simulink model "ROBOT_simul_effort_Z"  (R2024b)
settings: Solver=VariableStepAuto  StartTime=0.0  StopTime=5  RelTol=1e-3
undefined symbols (not defined in the file): a, ARRIERE_Defaut_sldprt, avant01_Defaut_sldprt, avant02_Defaut_sldprt, avant03_Defaut_sldprt, avant1_Defaut_sldprt, AXE, BASE_Defaut_sldprt, BIELLE, BIELLE_Defaut_sldprt, BRAS_Defaut_sldprt, bras_Defaut_sldprt, C_Realiste_sldprt, CABLE_Defaut_sldprt, cable_Defaut_sldprt, CACHE_Defaut_sldprt, CARTE, carte_Defaut_sldprt, CARTER, carter, CHC, CODEUR_Defaut_sldprt, cruciforme, cylindrique, deg, Drive, Fichiers, Fichiers_Matlab_sujetA, FIXATION, fixation_Defaut_sldprt, H, HEXAGONALE_Defaut_sldprt, joint_Defaut_sldprt, kg, m, M4, M4_Defaut_sldprt, manette1_Defaut_sldprt, manette2_Defaut_sldprt, MATLAB, Matlab, matlab_Defaut_sldprt, mm, modif, MOTEUR_Defaut_sldprt, N, NEZ_Defaut_sldprt, nom, palier, PARALLELOGRAMME_Defaut_sldprt, petite, plaque, rad, Ressort, Rondelle, ROTOR_Defaut_sldprt, s, SET, simple, socle_Defaut_sldprt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
libraries: sm_lib x463, fl_lib x45, nesl_utility x27, simulink x2
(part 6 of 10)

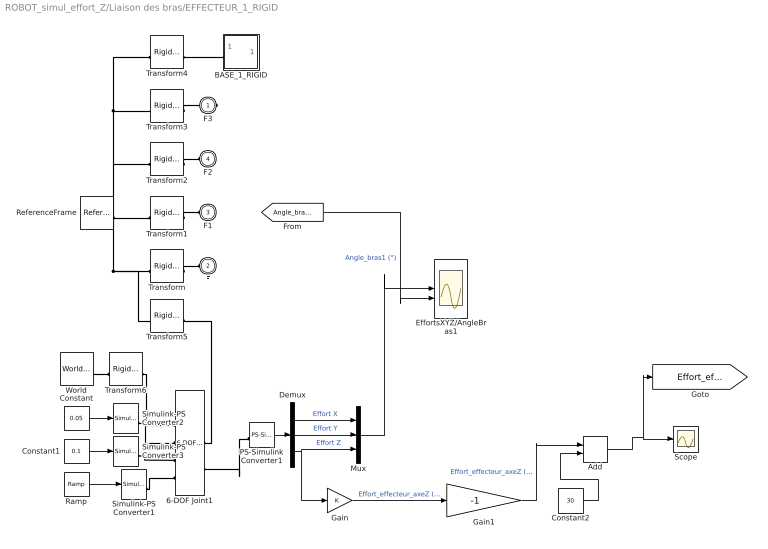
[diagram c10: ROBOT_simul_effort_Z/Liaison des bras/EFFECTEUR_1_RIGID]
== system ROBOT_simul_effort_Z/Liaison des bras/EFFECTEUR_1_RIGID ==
  6-DOF Joint1 : sm_lib/Joints/6-DOF Joint  JointMode=Normal  CompositeWrenchDir=FollowerOnBase  CompositeWrenchFrame=BaseFrame  SenseConstraintForce=off  SenseConstraintTorque=off  SenseTotalForce=on  SenseTotalTorque=off  PxPositionTargetSpecify=off  PxPositionTargetPriority=High  PxPositionTargetValue=0  PxPositionTargetValueUnits=m  PxVelocityTargetSpecify=off  PxVelocityTargetPriority=High  PxVelocityTargetValue=0  PxVelocityTargetValueUnits=m/s  PxEquilibriumPosition=0  PxEquilibriumPositionUnits=m  PxSpringStiffness=0  PxSpringStiffnessUnits=N/m  PxDampingCoefficient=0  PxDampingCoefficientUnits=N/(m/s)  PxLowerLimitSpecify=off  PxLowerLimitBound=-1  PxLowerLimitBoundUnits=m  PxLowerLimitStiffness=1e6  PxLowerLimitStiffnessUnits=N/m  PxLowerLimitDamping=1e3  PxLowerLimitDampingUnits=N/(m/s)  PxLowerLimitTransitionRegionWidth=1e-4  PxLowerLimitTransitionRegionWidthUnits=m  PxUpperLimitSpecify=off  PxUpperLimitBound=1  PxUpperLimitBoundUnits=m  PxUpperLimitStiffness=1e6  PxUpperLimitStiffnessUnits=N/m  PxUpperLimitDamping=1e3  PxUpperLimitDampingUnits=N/(m/s)  PxUpperLimitTransitionRegionWidth=1e-4  PxUpperLimitTransitionRegionWidthUnits=m  PxTorqueActuationMode=ComputedTorque  PxMotionActuationMode=InputMotion  PxSensePosition=off  PxSenseVelocity=off  PxSenseAcceleration=off  PxSenseTorqueForce=off  PxSenseLowerLimitTorqueForce=off  PxSenseUpperLimitTorqueForce=off  PyPositionTargetSpecify=off  PyPositionTargetPriority=High  PyPositionTargetValue=0  PyPositionTargetValueUnits=m  PyVelocityTargetSpecify=off  PyVelocityTargetPriority=High  PyVelocityTargetValue=0  PyVelocityTargetValueUnits=m/s  PyEquilibriumPosition=0  PyEquilibriumPositionUnits=m  PySpringStiffness=0  PySpringStiffnessUnits=N/m  PyDampingCoefficient=0  PyDampingCoefficientUnits=N/(m/s)  PyLowerLimitSpecify=off  PyLowerLimitBound=-1  PyLowerLimitBoundUnits=m  PyLowerLimitStiffness=1e6  PyLowerLimitStiffnessUnits=N/m  PyLowerLimitDamping=1e3  PyLowerLimitDampingUnits=N/(m/s)  PyLowerLimitTransitionRegionWidth=1e-4  PyLowerLimitTransitionRegionWidthUnits=m  PyUpperLimitSpecify=off  PyUpperLimitBound=1  PyUpperLimitBoundUnits=m  PyUpperLimitStiffness=1e6  PyUpperLimitStiffnessUnits=N/m  PyUpperLimitDamping=1e3  PyUpperLimitDampingUnits=N/(m/s)  PyUpperLimitTransitionRegionWidth=1e-4  PyUpperLimitTransitionRegionWidthUnits=m  PyTorqueActuationMode=ComputedTorque  PyMotionActuationMode=InputMotion  PySensePosition=off  PySenseVelocity=off  PySenseAcceleration=off  PySenseTorqueForce=off  PySenseLowerLimitTorqueForce=off  PySenseUpperLimitTorqueForce=off  PzPositionTargetSpecify=off  PzPositionTargetPriority=High  PzPositionTargetValue=0  PzPositionTargetValueUnits=m  PzVelocityTargetSpecify=off  PzVelocityTargetPriority=High  PzVelocityTargetValue=0  PzVelocityTargetValueUnits=m/s  PzEquilibriumPosition=0  PzEquilibriumPositionUnits=m  PzSpringStiffness=0  PzSpringStiffnessUnits=N/m  PzDampingCoefficient=0  PzDampingCoefficientUnits=N/(m/s)  PzLowerLimitSpecify=off  PzLowerLimitBound=-1  PzLowerLimitBoundUnits=m  PzLowerLimitStiffness=1e6  PzLowerLimitStiffnessUnits=N/m  PzLowerLimitDamping=1e3  PzLowerLimitDampingUnits=N/(m/s)  PzLowerLimitTransitionRegionWidth=1e-4  PzLowerLimitTransitionRegionWidthUnits=m  PzUpperLimitSpecify=off  PzUpperLimitBound=1  PzUpperLimitBoundUnits=m  PzUpperLimitStiffness=1e6  PzUpperLimitStiffnessUnits=N/m  PzUpperLimitDamping=1e3  PzUpperLimitDampingUnits=N/(m/s)  PzUpperLimitTransitionRegionWidth=1e-4  PzUpperLimitTransitionRegionWidthUnits=m  PzTorqueActuationMode=ComputedTorque  PzMotionActuationMode=InputMotion  PzSensePosition=off  PzSenseVelocity=off  PzSenseAcceleration=off  PzSenseTorqueForce=off  PzSenseLowerLimitTorqueForce=off  PzSenseUpperLimitTorqueForce=off  SphPositionTargetSpecify=off  SphPositionTargetPriority=High  SphPositionTargetRotationMethod=None  SphPositionTargetFollAlignAxisA=+X  SphPositionTargetBaseAlignAxisA=+Y  SphPositionTargetFollAlignAxisB=+Y  SphPositionTargetBaseAlignAxisB=+Z  SphPositionTargetRotationStandardAxis=+Z  SphPositionTargetRotationAngle=0.0  SphPositionTargetRotationAngleUnits=deg  SphPositionTargetRotationArbitraryAxis=[0 0 1]  SphPositionTargetRotationSequenceAxes=FollowerAxes  SphPositionTargetRotationSequence=XYX  SphPositionTargetRotationSequenceAngles=[0 0 0]  SphPositionTargetRotationSequenceAnglesUnits=deg  SphPositionTargetRotationMatrix=[1 0 0; 0 1 0; 0 0 1]  SphPositionTargetQuaternion=[1 0 0 0]  SphVelocityTargetSpecify=off  SphVelocityTargetPriority=High  SphVelocityTargetValue=[0 0 0]  SphVelocityTargetValueUnits=deg/s  SphVelocityTargetInFollowerFrame=on  SphEqPosRotationMethod=None  SphEqPosFollAlignAxisA=+X  SphEqPosBaseAlignAxisA=+Y  SphEqPosFollAlignAxisB=+Y  SphEqPosBaseAlignAxisB=+Z  SphEqPosRotationStandardAxis=+Z  SphEqPosRotationAngle=0.0  SphEqPosRotationAngleUnits=deg  SphEqPosRotationArbitraryAxis=[0 0 1]  SphEqPosRotationSequenceAxes=FollowerAxes  SphEqPosRotationSequence=XYX  SphEqPosRotationSequenceAngles=[0 0 0]  SphEqPosRotationSequenceAnglesUnits=deg  SphEqPosRotationMatrix=[1 0 0; 0 1 0; 0 0 1]  SphEqPosQuaternion=[1 0 0 0]  SphSpringStiffness=0  SphSpringStiffnessUnits=N*m/deg  SphDampingCoefficient=0  SphDampingCoefficientUnits=N*m/(deg/s)  SphLowerLimitSpecify=off  SphLowerLimitBound=15  SphLowerLimitBoundUnits=deg  SphLowerLimitStiffness=1e4  SphLowerLimitStiffnessUnits=N*m/deg  SphLowerLimitDamping=10  SphLowerLimitDampingUnits=N*m/(deg/s)  SphLowerLimitTransitionRegionWidth=0.1  SphLowerLimitTransitionRegionWidthUnits=deg  SphUpperLimitSpecify=off  SphUpperLimitBound=45  SphUpperLimitBoundUnits=deg  SphUpperLimitStiffness=1e4  SphUpperLimitStiffnessUnits=N*m/deg  SphUpperLimitDamping=10  SphUpperLimitDampingUnits=N*m/(deg/s)  SphUpperLimitTransitionRegionWidth=0.1  SphUpperLimitTransitionRegionWidthUnits=deg  SphTorqueActuationMode=NoTorque  SphActuateTorqueX=off  SphActuateTorqueY=off  SphActuateTorqueZ=off  SphActuateTorque=off  SphActuationFrame=BaseFrame  SphSensePosition=off  SphSenseVelocityX=off  SphSenseVelocityY=off  SphSenseVelocityZ=off  SphSenseVelocity=off  SphSenseAccelerationX=off  SphSenseAccelerationY=off  SphSenseAccelerationZ=off  SphSenseAcceleration=off  SphSenseLowerLimitTorqueMag=off  SphSenseUpperLimitTorqueMag=off  SphSensingFrame=BaseFrame
  Add : Sum
  BASE_1_RIGID : Subsystem
  Constant : Constant  Value=0.05
  Constant1 : Constant  Value=0.1
  Constant2 : Constant  Value=30
  Demux : Demux  Outputs=3
  EffortsXYZ/AngleBras1 : Scope  NumInputPorts=2
  Gain : Gain
  Gain1 : Gain  Gain=-1
  Mux : Mux  Inputs=3
  PS-Simulink Converter1 : nesl_utility/PS-Simulink Converter  PhysicalDomain=network_engine_domain  SubClassName=ps_output  LeftPortType=input  RightPortType=output  PseudoPeriodic=off  Frequencies=[]  VectorFormat=1-D array  Unit=1  AffineConversion=off
  Ramp : simulink/Sources/Ramp  slope=-0.022  start=0  InitialOutput=0.097
  ReferenceFrame : sm_lib/Frames and Transforms/Reference Frame
  Scope : Scope
  Simulink-PS Converter1 : nesl_utility/Simulink-PS Converter  PhysicalDomain=network_engine_domain  SubClassName=ps_input  LeftPortType=input  RightPortType=output  PseudoPeriodic=off  Frequencies=[]  NoiseDistribution=none  NoiseParameters=[]  Unit=m  AffineConversion=off  FilteringAndDerivatives=filter  SimscapeFilterOrder=2  InputFilterTimeConstant=0.0001  UdotUserProvided=1
  Simulink-PS Converter2 : nesl_utility/Simulink-PS Converter  PhysicalDomain=network_engine_domain  SubClassName=ps_input  LeftPortType=input  RightPortType=output  PseudoPeriodic=off  Frequencies=[]  NoiseDistribution=none  NoiseParameters=[]  Unit=m  AffineConversion=off  FilteringAndDerivatives=filter  SimscapeFilterOrder=2  InputFilterTimeConstant=0.0001  UdotUserProvided=1
  Simulink-PS Converter3 : nesl_utility/Simulink-PS Converter  PhysicalDomain=network_engine_domain  SubClassName=ps_input  LeftPortType=input  RightPortType=output  PseudoPeriodic=off  Frequencies=[]  NoiseDistribution=none  NoiseParameters=[]  Unit=m  AffineConversion=off  FilteringAndDerivatives=filter  SimscapeFilterOrder=2  InputFilterTimeConstant=0.0001  UdotUserProvided=1
  Transform : sm_lib/Frames and Transforms/Rigid Transform  RotationMethod=ArbitraryAxis  FollAlignAxisA=+X  BaseAlignAxisA=+Y  FollAlignAxisB=+Y  BaseAlignAxisB=+Z  RotationStandardAxis=+Z  RotationAngle=1.730474842144561  RotationAngleUnits=rad  RotationArbitraryAxis=[0.85183585180135124 0.37038876979862273 0.37038876979861218]  RotationSequenceAxes=FollowerAxes  RotationSequence=XYX  RotationSequenceAngles=[0 0 0]  RotationSequenceAnglesUnits=deg  RotationMatrix=[1 0 0; 0 1 0; 0 0 1]  Quaternion=[1 0 0 0]  TranslationMethod=Cartesian  TranslationCartesianOffset=[-87.428721422199686 114.78475141038592 178.68957730413138]  TranslationCartesianOffsetUnits=mm  TranslationStandardAxis=+Z  TranslationStandardOffset=0  TranslationStandardOffsetUnits=mm  TranslationROffset=0  TranslationROffsetUnits=m  TranslationThetaOffset=0  TranslationThetaOffsetUnits=deg  TranslationZOffset=0  TranslationZOffsetUnits=m
  Transform1 : sm_lib/Frames and Transforms/Rigid Transform  RotationMethod=ArbitraryAxis  FollAlignAxisA=+X  BaseAlignAxisA=+Y  FollAlignAxisB=+Y  BaseAlignAxisB=+Z  RotationStandardAxis=+Z  RotationAngle=2.2299847707569485  RotationAngleUnits=rad  RotationArbitraryAxis=[-0.6163079985177109 -0.49023351775065482 -0.61630799851771478]  RotationSequenceAxes=FollowerAxes  RotationSequence=XYX  RotationSequenceAngles=[0 0 0]  RotationSequenceAnglesUnits=deg  RotationMatrix=[1 0 0; 0 1 0; 0 0 1]  Quaternion=[1 0 0 0]  TranslationMethod=Cartesian  TranslationCartesianOffset=[-45.597843791303056 49.588932155076364 178.68957730412913]  TranslationCartesianOffsetUnits=mm  TranslationStandardAxis=+Z  TranslationStandardOffset=0  TranslationStandardOffsetUnits=mm  TranslationROffset=0  TranslationROffsetUnits=m  TranslationThetaOffset=0  TranslationThetaOffsetUnits=deg  TranslationZOffset=0  TranslationZOffsetUnits=m
  Transform2 : sm_lib/Frames and Transforms/Rigid Transform  RotationMethod=ArbitraryAxis  FollAlignAxisA=+X  BaseAlignAxisA=+Y  FollAlignAxisB=+Y  BaseAlignAxisB=+Z  RotationStandardAxis=+Z  RotationAngle=2.2733724201793901  RotationAngleUnits=rad  RotationArbitraryAxis=[-0.46360505726599749 -0.62652627673442052 0.62652627673442052]  RotationSequenceAxes=FollowerAxes  RotationSequence=XYX  RotationSequenceAngles=[0 0 0]  RotationSequenceAnglesUnits=deg  RotationMatrix=[1 0 0; 0 1 0; 0 0 1]  Quaternion=[1 0 0 0]  TranslationMethod=Cartesian  TranslationCartesianOffset=[-11.168668790429919 124.06200864616406 178.68957730412961]  TranslationCartesianOffsetUnits=mm  TranslationStandardAxis=+Z  TranslationStandardOffset=0  TranslationStandardOffsetUnits=mm  TranslationROffset=0  TranslationROffsetUnits=m  TranslationThetaOffset=0  TranslationThetaOffsetUnits=deg  TranslationZOffset=0  TranslationZOffsetUnits=m
  Transform3 : sm_lib/Frames and Transforms/Rigid Transform  RotationMethod=ArbitraryAxis  FollAlignAxisA=+X  BaseAlignAxisA=+Y  FollAlignAxisB=+Y  BaseAlignAxisB=+Z  RotationStandardAxis=+Z  RotationAngle=pi  RotationAngleUnits=rad  RotationArbitraryAxis=[-1 0 0]  RotationSequenceAxes=FollowerAxes  RotationSequence=XYX  RotationSequenceAngles=[0 0 0]  RotationSequenceAnglesUnits=deg  RotationMatrix=[1 0 0; 0 1 0; 0 0 1]  Quaternion=[1 0 0 0]  TranslationMethod=Cartesian  TranslationCartesianOffset=[-18.52 120.86 192.69]  TranslationCartesianOffsetUnits=mm  TranslationStandardAxis=+Z  TranslationStandardOffset=0  TranslationStandardOffsetUnits=mm  TranslationROffset=0  TranslationROffsetUnits=m  TranslationThetaOffset=0  TranslationThetaOffsetUnits=deg  TranslationZOffset=0  TranslationZOffsetUnits=m
  Transform4 : sm_lib/Frames and Transforms/Rigid Transform  RotationMethod=ArbitraryAxis  FollAlignAxisA=+X  BaseAlignAxisA=+Y  FollAlignAxisB=+Y  BaseAlignAxisB=+Z  RotationStandardAxis=+Z  RotationAngle=0.13705421065001749  RotationAngleUnits=rad  RotationArbitraryAxis=[5.1539164000577042e-14 1.7402105179219416e-14 -1]  RotationSequenceAxes=FollowerAxes  RotationSequence=XYX  RotationSequenceAngles=[0 0 0]  RotationSequenceAnglesUnits=deg  RotationMatrix=[1 0 0; 0 1 0; 0 0 1]  Quaternion=[1 0 0 0]  TranslationMethod=Cartesian  TranslationCartesianOffset=[-48.809383170568495 97.91432372411964 187.1895773041295]  TranslationCartesianOffsetUnits=mm  TranslationStandardAxis=+Z  TranslationStandardOffset=0  TranslationStandardOffsetUnits=mm  TranslationROffset=0  TranslationROffsetUnits=m  TranslationThetaOffset=0  TranslationThetaOffsetUnits=deg  TranslationZOffset=0  TranslationZOffsetUnits=m
  Transform5 : sm_lib/Frames and Transforms/Rigid Transform  RotationMethod=ArbitraryAxis  FollAlignAxisA=+X  BaseAlignAxisA=+Y  FollAlignAxisB=+Y  BaseAlignAxisB=+Z  RotationStandardAxis=+Z  RotationAngle=pi  RotationAngleUnits=rad  RotationArbitraryAxis=[-1 0 0]  RotationSequenceAxes=FollowerAxes  RotationSequence=XYX  RotationSequenceAngles=[0 0 0]  RotationSequenceAnglesUnits=deg  RotationMatrix=[1 0 0; 0 1 0; 0 0 1]  Quaternion=[1 0 0 0]  TranslationMethod=Cartesian  TranslationCartesianOffset=[-18.52 120.86 192.69]  TranslationCartesianOffsetUnits=mm  TranslationStandardAxis=+Z  TranslationStandardOffset=0  TranslationStandardOffsetUnits=mm  TranslationROffset=0  TranslationROffsetUnits=m  TranslationThetaOffset=0  TranslationThetaOffsetUnits=deg  TranslationZOffset=0  TranslationZOffsetUnits=m
  Transform6 : sm_lib/Frames and Transforms/Rigid Transform  RotationMethod=ArbitraryAxis  FollAlignAxisA=+X  BaseAlignAxisA=+Y  FollAlignAxisB=+Y  BaseAlignAxisB=+Z  RotationStandardAxis=+Z  RotationAngle=pi  RotationAngleUnits=rad  RotationArbitraryAxis=[-1 0 0]  RotationSequenceAxes=FollowerAxes  RotationSequence=XYX  RotationSequenceAngles=[0 0 0]  RotationSequenceAnglesUnits=deg  RotationMatrix=[1 0 0; 0 1 0; 0 0 1]  Quaternion=[1 0 0 0]  TranslationMethod=Cartesian  TranslationCartesianOffset=[-18.52 120.86 192.69]  TranslationCartesianOffsetUnits=mm  TranslationStandardAxis=+Z  TranslationStandardOffset=0  TranslationStandardOffsetUnits=mm  TranslationROffset=0  TranslationROffsetUnits=m  TranslationThetaOffset=0  TranslationThetaOffsetUnits=deg  TranslationZOffset=0  TranslationZOffsetUnits=m
  World : sm_lib/Frames and Transforms/World Frame
  F3 : PMIOPort  Side=Right
  F : PMIOPort  Port=2  Side=Left
  F1 : PMIOPort  Port=3  Side=Left
  F2 : PMIOPort  Port=4  Side=Left
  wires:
  Ramp/1 -> Simulink-PS Converter1/1
  Demux/3 -> Gain/1, Mux/3  "Effort Z"
  Constant/1 -> Simulink-PS Converter2/1
  Constant1/1 -> Simulink-PS Converter3/1
  [Angle_bras1] -> EffortsXYZ/AngleBras1/2  "Angle_bras1 (°)"
  Mux/1 -> EffortsXYZ/AngleBras1/1
  Demux/1 -> Mux/1  "Effort X"
  Demux/2 -> Mux/2  "Effort Y"
  PS-Simulink Converter1/1 -> Demux/1
  Gain/1 -> Gain1/1  "Effort_effecteur_axeZ (N)"
  Gain1/1 -> Add/1  "Effort_effecteur_axeZ (N)"
  Add/1 -> [Effort_effecteur], Scope/1
  Constant2/1 -> Add/2
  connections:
  ReferenceFrame/RConn1 -- Transform5/LConn1 -- Transform/LConn1 -- Transform1/LConn1 -- Transform2/LConn1 -- Transform3/LConn1 -- Transform4/LConn1
  Transform/RConn1 -- F/RConn1
  Transform1/RConn1 -- F1/RConn1
  Transform2/RConn1 -- F2/RConn1
  Transform3/RConn1 -- F3/RConn1
  BASE_1_RIGID/LConn1 -- Transform4/RConn1
  Simulink-PS Converter1/RConn1 -- 6-DOF Joint1/LConn4
  6-DOF Joint1/RConn1 -- Transform5/RConn1
  Transform6/RConn1 -- 6-DOF Joint1/LConn1
  World/RConn1 -- Transform6/LConn1
  Simulink-PS Converter2/RConn1 -- 6-DOF Joint1/LConn2
  Simulink-PS Converter3/RConn1 -- 6-DOF Joint1/LConn3
  PS-Simulink Converter1/LConn1 -- 6-DOF Joint1/RConn2

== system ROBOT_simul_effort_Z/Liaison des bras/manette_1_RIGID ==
  ReferenceFrame : sm_lib/Frames and Transforms/Reference Frame
  Transform : sm_lib/Frames and Transforms/Rigid Transform  RotationMethod=ArbitraryAxis  FollAlignAxisA=+X  BaseAlignAxisA=+Y  FollAlignAxisB=+Y  BaseAlignAxisB=+Z  RotationStandardAxis=+Z  RotationAngle=2.2920311904365782  RotationAngleUnits=rad  RotationArbitraryAxis=[0.63063758405056181 -0.45231899713116352 0.63063758405056158]  RotationSequenceAxes=FollowerAxes  RotationSequence=XYX  RotationSequenceAngles=[0 0 0]  RotationSequenceAnglesUnits=deg  RotationMatrix=[1 0 0; 0 1 0; 0 0 1]  Quaternion=[1 0 0 0]  TranslationMethod=Cartesian  TranslationCartesianOffset=[-33.84478008900291 22.436374240911583 2.2257143640758983]  TranslationCartesianOffsetUnits=mm  TranslationStandardAxis=+Z  TranslationStandardOffset=0  TranslationStandardOffsetUnits=mm  TranslationROffset=0  TranslationROffsetUnits=m  TranslationThetaOffset=0  TranslationThetaOffsetUnits=deg  TranslationZOffset=0  TranslationZOffsetUnits=m
  Transform1 : sm_lib/Frames and Transforms/Rigid Transform  RotationMethod=ArbitraryAxis  FollAlignAxisA=+X  BaseAlignAxisA=+Y  FollAlignAxisB=+Y  BaseAlignAxisB=+Z  RotationStandardAxis=+Z  RotationAngle=3.1415926535897931  RotationAngleUnits=rad  RotationArbitraryAxis=[-0.15005935073897111 0.98867699035417955 -3.0703282687218866e-18]  RotationSequenceAxes=FollowerAxes  RotationSequence=XYX  RotationSequenceAngles=[0 0 0]  RotationSequenceAnglesUnits=deg  RotationMatrix=[1 0 0; 0 1 0; 0 0 1]  Quaternion=[1 0 0 0]  TranslationMethod=Cartesian  TranslationCartesianOffset=[-57.010083199545775 -8.8196659542755462 4.7257143640759303]  TranslationCartesianOffsetUnits=mm  TranslationStandardAxis=+Z  TranslationStandardOffset=0  TranslationStandardOffsetUnits=mm  TranslationROffset=0  TranslationROffsetUnits=m  TranslationThetaOffset=0  TranslationThetaOffsetUnits=deg  TranslationZOffset=0  TranslationZOffsetUnits=m
  Transform2 : sm_lib/Frames and Transforms/Rigid Transform  RotationMethod=None  FollAlignAxisA=+X  BaseAlignAxisA=+Y  FollAlignAxisB=+Y  BaseAlignAxisB=+Z  RotationStandardAxis=+Z  RotationAngle=0  RotationAngleUnits=deg  RotationArbitraryAxis=[0 0 1]  RotationSequenceAxes=FollowerAxes  RotationSequence=XYX  RotationSequenceAngles=[0 0 0]  RotationSequenceAnglesUnits=deg  RotationMatrix=[1 0 0; 0 1 0; 0 0 1]  Quaternion=[1 0 0 0]  TranslationMethod=Cartesian  TranslationCartesianOffset=[-33.322737031332075 20.894129352085105 2.2257143640758983]  TranslationCartesianOffsetUnits=mm  TranslationStandardAxis=+Z  TranslationStandardOffset=0  TranslationStandardOffsetUnits=mm  TranslationROffset=0  TranslationROffsetUnits=m  TranslationThetaOffset=0  TranslationThetaOffsetUnits=deg  TranslationZOffset=0  TranslationZOffsetUnits=m
  manette1_1_RIGID : Subsystem
  F : PMIOPort  Side=Right
  F1 : PMIOPort  Port=2  Side=Left
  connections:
  Transform/LConn1 -- ReferenceFrame/RConn1 -- Transform1/LConn1 -- Transform2/LConn1
  Transform/RConn1 -- F/RConn1
  Transform1/RConn1 -- F1/RConn1
  Transform2/RConn1 -- manette1_1_RIGID/LConn1

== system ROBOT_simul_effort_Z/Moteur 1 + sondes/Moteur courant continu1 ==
  note: Kv = 1.18e-1
  Frottement : fl_lib/Mechanical/Rotational Elements/Rotational Friction  brkwy_trq=2.43e-3 N*m  brkwy_vel=0.030296 rad/s  Col_trq=2.43e-3 N*m  visc_coef=2e-6 N*m/(rad/s)  w_specify=off  w_priority=None  w=0 rad/s  w_nominal_specify=off  w_nominal_value=1  w_nominal_unit=rad/s  t_specify=off  t_priority=None  t=0 N*m  t_nominal_specify=off  t_nominal_value=1  t_nominal_unit=N*m
  Inductance induit 35mH : fl_lib/Electrical/Electrical Elements/Inductor  l=35 mH  r=0 Ohm  g=1e-09 1/Ohm  i_specify=off  i_priority=None  i=0 A  i_nominal_specify=off  i_nominal_value=1  i_nominal_unit=A  v_specify=off  v_priority=None  v=0 V  v_nominal_specify=off  v_nominal_value=1  v_nominal_unit=V  i_L_specify=on  i_L_priority=High  i_L=0 A  i_L_nominal_specify=off  i_L_nominal_value=1  i_L_nominal_unit=A
  Inertie Je 10e-6 : fl_lib/Mechanical/Rotational Elements/Inertia  inertia=10e-6 kg*m^2  num_ports=foundation.enum.numPorts2.one  w_specify=on  w_priority=High  w=0 rad/s  w_nominal_specify=off  w_nominal_value=1  w_nominal_unit=rad/s  t_specify=off  t_priority=None  t=0 N*m  t_nominal_specify=off  t_nominal_value=1  t_nominal_unit=N*m
  Moteur parfait : fl_lib/Electrical/Electrical Elements/Rotational Electromechanical Converter  K=1.18e-1 V/(rad/s)  i_specify=off  i_priority=None  i=0 A  i_nominal_specify=off  i_nominal_value=1  i_nominal_unit=A  v_specify=off  v_priority=None  v=0 V  v_nominal_specify=off  v_nominal_value=1  v_nominal_unit=V  t_specify=off  t_priority=None  t=0 N*m  t_nominal_specify=off  t_nominal_value=1  t_nominal_unit=N*m  w_specify=off  w_priority=None  w=0 rad/s  w_nominal_specify=off  w_nominal_value=1  w_nominal_unit=rad/s
  Rinduit 38 Ohms : fl_lib/Electrical/Electrical Elements/Resistor  Tag=Factory Generic  R=38 Ohm  i_specify=off  i_priority=None  i=0 A  i_nominal_specify=off  i_nominal_value=1  i_nominal_unit=A  v_specify=off  v_priority=None  v=0 V  v_nominal_specify=off  v_nominal_value=1  v_nominal_unit=V
  V+ : PMIOPort  Side=Left
  R : PMIOPort  Port=2  Side=Right
  C : PMIOPort  Port=3  Side=Right
  V- : PMIOPort  Port=4  Side=Left
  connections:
  C/RConn1 -- Moteur parfait/RConn2 -- Frottement/RConn1
  R/RConn1 -- Inertie Je 10e-6/LConn1 -- Moteur parfait/LConn2 -- Frottement/LConn1
  Inductance induit 35mH/LConn1 -- Rinduit 38 Ohms/RConn1
  Rinduit 38 Ohms/LConn1 -- V+/RConn1
  V-/RConn1 -- Moteur parfait/RConn1
  Moteur parfait/LConn1 -- Inductance induit 35mH/RConn1

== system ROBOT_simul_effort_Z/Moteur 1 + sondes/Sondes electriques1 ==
  " Conv i" : nesl_utility/PS-Simulink Converter  PhysicalDomain=network_engine_domain  SubClassName=ps_output  LeftPortType=input  RightPortType=output  PseudoPeriodic=off  Frequencies=[]  VectorFormat=1-D array  Unit=1  AffineConversion=off
  " Conv v" : nesl_utility/PS-Simulink Converter  PhysicalDomain=network_engine_domain  SubClassName=ps_output  LeftPortType=input  RightPortType=output  PseudoPeriodic=off  Frequencies=[]  VectorFormat=1-D array  Unit=1  AffineConversion=off
  Bras1 : Scope  NumInputPorts=2
  Invers signe : Gain
  Invers signe1 : Gain
  Sonde_I : fl_lib/Electrical/Electrical Sensors/Current Sensor
  Sonde_U : fl_lib/Electrical/Electrical Sensors/Voltage Sensor
  Conn1 : PMIOPort  Side=Left
  Conn2 : PMIOPort  Port=2  Side=Right
  Conn3 : PMIOPort  Port=3  Side=Right
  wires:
  [i] -> Invers signe1/1  "Imoteur1"
  [u] -> Invers signe/1  "Umoteur1"
  " Conv i"/1 -> [i]
  " Conv v"/1 -> [u]
  Invers signe/1 -> Bras1/1  "Umoteur1(V)"
  Invers signe1/1 -> Bras1/2  "Imoteur1(A)"
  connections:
  Conn3/RConn1 -- Sonde_U/RConn2
  Conn2/RConn1 -- Sonde_I/RConn2
  Sonde_I/LConn1 -- Sonde_U/LConn1 -- Conn1/RConn1
  Sonde_U/RConn1 -- " Conv v"/LConn1
  Sonde_I/RConn1 -- " Conv i"/LConn1

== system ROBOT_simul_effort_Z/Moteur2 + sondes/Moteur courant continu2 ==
  note: Kv = 1.18e-1
  Frottement : fl_lib/Mechanical/Rotational Elements/Rotational Friction  brkwy_trq=2.43e-3 N*m  brkwy_vel=0.030296 rad/s  Col_trq=2.43e-3 N*m  visc_coef=2e-6 N*m/(rad/s)  w_specify=off  w_priority=None  w=0 rad/s  w_nominal_specify=off  w_nominal_value=1  w_nominal_unit=rad/s  t_specify=off  t_priority=None  t=0 N*m  t_nominal_specify=off  t_nominal_value=1  t_nominal_unit=N*m
  Inductance induit 35mH : fl_lib/Electrical/Electrical Elements/Inductor  l=35 mH  r=0 Ohm  g=1e-09 1/Ohm  i_specify=off  i_priority=None  i=0 A  i_nominal_specify=off  i_nominal_value=1  i_nominal_unit=A  v_specify=off  v_priority=None  v=0 V  v_nominal_specify=off  v_nominal_value=1  v_nominal_unit=V  i_L_specify=on  i_L_priority=High  i_L=0 A  i_L_nominal_specify=off  i_L_nominal_value=1  i_L_nominal_unit=A
  Inertie Je 10e-6 : fl_lib/Mechanical/Rotational Elements/Inertia  inertia=10e-6 kg*m^2  num_ports=foundation.enum.numPorts2.one  w_specify=on  w_priority=High  w=0 rad/s  w_nominal_specify=off  w_nominal_value=1  w_nominal_unit=rad/s  t_specify=off  t_priority=None  t=0 N*m  t_nominal_specify=off  t_nominal_value=1  t_nominal_unit=N*m
  Moteur parfait : fl_lib/Electrical/Electrical Elements/Rotational Electromechanical Converter  K=1.18e-1 V/(rad/s)  i_specify=off  i_priority=None  i=0 A  i_nominal_specify=off  i_nominal_value=1  i_nominal_unit=A  v_specify=off  v_priority=None  v=0 V  v_nominal_specify=off  v_nominal_value=1  v_nominal_unit=V  t_specify=off  t_priority=None  t=0 N*m  t_nominal_specify=off  t_nominal_value=1  t_nominal_unit=N*m  w_specify=off  w_priority=None  w=0 rad/s  w_nominal_specify=off  w_nominal_value=1  w_nominal_unit=rad/s
  Rinduit 38 Ohms : fl_lib/Electrical/Electrical Elements/Resistor  Tag=Factory Generic  R=38 Ohm  i_specify=off  i_priority=None  i=0 A  i_nominal_specify=off  i_nominal_value=1  i_nominal_unit=A  v_specify=off  v_priority=None  v=0 V  v_nominal_specify=off  v_nominal_value=1  v_nominal_unit=V
  V+ : PMIOPort  Side=Left
  R : PMIOPort  Port=2  Side=Right
  C : PMIOPort  Port=3  Side=Right
  V- : PMIOPort  Port=4  Side=Left
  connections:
  Moteur parfait/LConn1 -- Inductance induit 35mH/RConn1
  V-/RConn1 -- Moteur parfait/RConn1
  Rinduit 38 Ohms/LConn1 -- V+/RConn1
  Inductance induit 35mH/LConn1 -- Rinduit 38 Ohms/RConn1
  Frottement/LConn1 -- Moteur parfait/LConn2 -- Inertie Je 10e-6/LConn1 -- R/RConn1
  Frottement/RConn1 -- Moteur parfait/RConn2 -- C/RConn1

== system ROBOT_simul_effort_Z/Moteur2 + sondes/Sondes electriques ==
  " Conv i" : nesl_utility/PS-Simulink Converter  PhysicalDomain=network_engine_domain  SubClassName=ps_output  LeftPortType=input  RightPortType=output  PseudoPeriodic=off  Frequencies=[]  VectorFormat=1-D array  Unit=1  AffineConversion=off
  " Conv v" : nesl_utility/PS-Simulink Converter  PhysicalDomain=network_engine_domain  SubClassName=ps_output  LeftPortType=input  RightPortType=output  PseudoPeriodic=off  Frequencies=[]  VectorFormat=1-D array  Unit=1  AffineConversion=off
  Bras2 : Scope  NumInputPorts=2
  Sonde_I : fl_lib/Electrical/Electrical Sensors/Current Sensor
  Sonde_U : fl_lib/Electrical/Electrical Sensors/Voltage Sensor
  Conn1 : PMIOPort  Side=Left
  Conn2 : PMIOPort  Port=2  Side=Right
  Conn3 : PMIOPort  Port=3  Side=Right
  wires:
  " Conv v"/1 -> [u]
  " Conv i"/1 -> [i]
  [u] -> Bras2/1  "Umoteur2"
  [i] -> Bras2/2  "Imoteur2"
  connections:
  Sonde_I/RConn1 -- " Conv i"/LConn1
  Sonde_U/RConn1 -- " Conv v"/LConn1
  Conn1/RConn1 -- Sonde_U/LConn1 -- Sonde_I/LConn1
  Conn2/RConn1 -- Sonde_I/RConn2
  Conn3/RConn1 -- Sonde_U/RConn2

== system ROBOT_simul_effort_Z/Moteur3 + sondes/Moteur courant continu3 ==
  note: Kv = 1.18e-1
  Frottement : fl_lib/Mechanical/Rotational Elements/Rotational Friction  brkwy_trq=2.43e-3 N*m  brkwy_vel=0.030296 rad/s  Col_trq=2.43e-3 N*m  visc_coef=2e-6 N*m/(rad/s)  w_specify=off  w_priority=None  w=0 rad/s  w_nominal_specify=off  w_nominal_value=1  w_nominal_unit=rad/s  t_specify=off  t_priority=None  t=0 N*m  t_nominal_specify=off  t_nominal_value=1  t_nominal_unit=N*m
  Inductance induit 35mH : fl_lib/Electrical/Electrical Elements/Inductor  l=35 mH  r=0 Ohm  g=1e-09 1/Ohm  i_specify=off  i_priority=None  i=0 A  i_nominal_specify=off  i_nominal_value=1  i_nominal_unit=A  v_specify=off  v_priority=None  v=0 V  v_nominal_specify=off  v_nominal_value=1  v_nominal_unit=V  i_L_specify=on  i_L_priority=High  i_L=0 A  i_L_nominal_specify=off  i_L_nominal_value=1  i_L_nominal_unit=A
  Inertie Je 10e-6 : fl_lib/Mechanical/Rotational Elements/Inertia  inertia=10e-6 kg*m^2  num_ports=foundation.enum.numPorts2.one  w_specify=on  w_priority=High  w=0 rad/s  w_nominal_specify=off  w_nominal_value=1  w_nominal_unit=rad/s  t_specify=off  t_priority=None  t=0 N*m  t_nominal_specify=off  t_nominal_value=1  t_nominal_unit=N*m
  Moteur parfait : fl_lib/Electrical/Electrical Elements/Rotational Electromechanical Converter  K=1.18e-1 V/(rad/s)  i_specify=off  i_priority=None  i=0 A  i_nominal_specify=off  i_nominal_value=1  i_nominal_unit=A  v_specify=off  v_priority=None  v=0 V  v_nominal_specify=off  v_nominal_value=1  v_nominal_unit=V  t_specify=off  t_priority=None  t=0 N*m  t_nominal_specify=off  t_nominal_value=1  t_nominal_unit=N*m  w_specify=off  w_priority=None  w=0 rad/s  w_nominal_specify=off  w_nominal_value=1  w_nominal_unit=rad/s
  Rinduit 38 Ohms : fl_lib/Electrical/Electrical Elements/Resistor  Tag=Factory Generic  R=38 Ohm  i_specify=off  i_priority=None  i=0 A  i_nominal_specify=off  i_nominal_value=1  i_nominal_unit=A  v_specify=off  v_priority=None  v=0 V  v_nominal_specify=off  v_nominal_value=1  v_nominal_unit=V
  V+ : PMIOPort  Side=Left
  R : PMIOPort  Port=2  Side=Right
  C : PMIOPort  Port=3  Side=Right
  V- : PMIOPort  Port=4  Side=Left
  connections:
  Moteur parfait/LConn1 -- Inductance induit 35mH/RConn1
  V-/RConn1 -- Moteur parfait/RConn1
  Rinduit 38 Ohms/LConn1 -- V+/RConn1
  Inductance induit 35mH/LConn1 -- Rinduit 38 Ohms/RConn1
  Frottement/LConn1 -- Moteur parfait/LConn2 -- Inertie Je 10e-6/LConn1 -- R/RConn1
  Frottement/RConn1 -- Moteur parfait/RConn2 -- C/RConn1

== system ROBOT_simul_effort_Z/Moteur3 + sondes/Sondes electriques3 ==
  " Conv i" : nesl_utility/PS-Simulink Converter  PhysicalDomain=network_engine_domain  SubClassName=ps_output  LeftPortType=input  RightPortType=output  PseudoPeriodic=off  Frequencies=[]  VectorFormat=1-D array  Unit=1  AffineConversion=off
  " Conv v" : nesl_utility/PS-Simulink Converter  PhysicalDomain=network_engine_domain  SubClassName=ps_output  LeftPortType=input  RightPortType=output  PseudoPeriodic=off  Frequencies=[]  VectorFormat=1-D array  Unit=1  AffineConversion=off
  Bras3 : Scope  NumInputPorts=2
  Sonde_I : fl_lib/Electrical/Electrical Sensors/Current Sensor
  Sonde_U : fl_lib/Electrical/Electrical Sensors/Voltage Sensor
  Conn1 : PMIOPort  Side=Left
  Conn2 : PMIOPort  Port=2  Side=Right
  Conn3 : PMIOPort  Port=3  Side=Right
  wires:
  " Conv v"/1 -> [u]
  " Conv i"/1 -> [i]
  [u] -> Bras3/1  "Umoteur3"
  [i] -> Bras3/2  "Imoteur3"
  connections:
  Sonde_I/RConn1 -- " Conv i"/LConn1
  Sonde_U/RConn1 -- " Conv v"/LConn1
  Conn1/RConn1 -- Sonde_U/LConn1 -- Sonde_I/LConn1
  Conn2/RConn1 -- Sonde_I/RConn2
  Conn3/RConn1 -- Sonde_U/RConn2

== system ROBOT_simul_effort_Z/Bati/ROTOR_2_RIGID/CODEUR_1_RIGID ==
  ReferenceFrame : sm_lib/Frames and Transforms/Reference Frame
  Solid : sm_lib/Body Elements/File Solid  ExtGeomFileName=/MATLAB Drive/Fichiers_Matlab_sujetA/Fichiers Matlab/STL/CODEUR_Defaut_sldprt.STL  UnitType=Custom  ExtGeomFileUnits=mm  StepReaderType=HEX  ExportConvexHullGeometry=off  InertiaType=Custom  BasedOnType=Density  Density=1000  DensityUnits=kg/(m^3)  Mass=0.0064318274490095598  MassUnits=kg  CenterOfMass=[0 6.0527709306807029 -0.1964144966449296]  CenterOfMassUnits=mm  MomentsOfInertia=[0.92812714377460337 1.2443807481520079 0.93469179577802664]  MomentsOfInertiaUnits=kg*mm^2  ProductsOfInertia=[0.0063987198741970201 0 0]  ProductsOfInertiaUnits=kg*mm^2  GraphicType=FromGeometry  MarkerShape=Sphere  MarkerSize=10  GraphicVisPropType=SimpleVisualProperties  GraphicDiffuseColor=[0.2 1.0 0.2]  GraphicOpacity=1  GraphicSpecularColor=[0.5 0.5 0.5 1.0]  GraphicAmbientColor=[0.15 0.15 0.15 1.0]  GraphicEmissiveColor=[0.0 0.0 0.0 1.0]  GraphicShininess=75  DoExposeReferenceFrame=on  SerializedFrames=<Frames/>
  F : PMIOPort  Side=Left
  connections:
  Solid/RConn1 -- ReferenceFrame/RConn1 -- F/RConn1

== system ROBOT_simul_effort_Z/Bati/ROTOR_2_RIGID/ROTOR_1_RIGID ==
  ReferenceFrame : sm_lib/Frames and Transforms/Reference Frame
  Solid : sm_lib/Body Elements/File Solid  ExtGeomFileName=/MATLAB Drive/Fichiers_Matlab_sujetA/Fichiers Matlab/STL/ROTOR_Defaut_sldprt.STL  UnitType=Custom  ExtGeomFileUnits=mm  StepReaderType=HEX  ExportConvexHullGeometry=off  InertiaType=Custom  BasedOnType=Density  Density=1000  DensityUnits=kg/(m^3)  Mass=0.07643998420030651  MassUnits=kg  CenterOfMass=[0 30.928341108151987 -0.0018262913863015125]  CenterOfMassUnits=mm  MomentsOfInertia=[14.640748377051393 9.6696912582654697 14.640902193857929]  MomentsOfInertiaUnits=kg*mm^2  ProductsOfInertia=[0.0065014820412302417 0 0]  ProductsOfInertiaUnits=kg*mm^2  GraphicType=FromGeometry  MarkerShape=Sphere  MarkerSize=10  GraphicVisPropType=SimpleVisualProperties  GraphicDiffuseColor=[0.53725490196078429 0.34901960784313724 0.33725490196078434]  GraphicOpacity=1  GraphicSpecularColor=[0.5 0.5 0.5 1.0]  GraphicAmbientColor=[0.15 0.15 0.15 1.0]  GraphicEmissiveColor=[0.0 0.0 0.0 1.0]  GraphicShininess=75  DoExposeReferenceFrame=on  SerializedFrames=<Frames/>
  F : PMIOPort  Side=Left
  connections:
  Solid/RConn1 -- ReferenceFrame/RConn1 -- F/RConn1

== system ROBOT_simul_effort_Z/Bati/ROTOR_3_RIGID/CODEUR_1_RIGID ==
  ReferenceFrame : sm_lib/Frames and Transforms/Reference Frame
  Solid : sm_lib/Body Elements/File Solid  ExtGeomFileName=/MATLAB Drive/Fichiers_Matlab_sujetA/Fichiers Matlab/STL/CODEUR_Defaut_sldprt.STL  UnitType=Custom  ExtGeomFileUnits=mm  StepReaderType=HEX  ExportConvexHullGeometry=off  InertiaType=Custom  BasedOnType=Density  Density=1000  DensityUnits=kg/(m^3)  Mass=0.0064318274490095598  MassUnits=kg  CenterOfMass=[0 6.0527709306807029 -0.1964144966449296]  CenterOfMassUnits=mm  MomentsOfInertia=[0.92812714377460337 1.2443807481520079 0.93469179577802664]  MomentsOfInertiaUnits=kg*mm^2  ProductsOfInertia=[0.0063987198741970201 0 0]  ProductsOfInertiaUnits=kg*mm^2  GraphicType=FromGeometry  MarkerShape=Sphere  MarkerSize=10  GraphicVisPropType=SimpleVisualProperties  GraphicDiffuseColor=[0.792156862745098 0.81960784313725488 0.93333333333333335]  GraphicOpacity=1  GraphicSpecularColor=[0.5 0.5 0.5 1.0]  GraphicAmbientColor=[0.15 0.15 0.15 1.0]  GraphicEmissiveColor=[0.0 0.0 0.0 1.0]  GraphicShininess=75  DoExposeReferenceFrame=on  SerializedFrames=<Frames/>
  F : PMIOPort  Side=Left
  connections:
  Solid/RConn1 -- ReferenceFrame/RConn1 -- F/RConn1

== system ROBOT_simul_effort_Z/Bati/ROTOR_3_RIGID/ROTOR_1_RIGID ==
  ReferenceFrame : sm_lib/Frames and Transforms/Reference Frame
  Solid : sm_lib/Body Elements/File Solid  ExtGeomFileName=/MATLAB Drive/Fichiers_Matlab_sujetA/Fichiers Matlab/STL/ROTOR_Defaut_sldprt.STL  UnitType=Custom  ExtGeomFileUnits=mm  StepReaderType=HEX  ExportConvexHullGeometry=off  InertiaType=Custom  BasedOnType=Density  Density=1000  DensityUnits=kg/(m^3)  Mass=0.07643998420030651  MassUnits=kg  CenterOfMass=[0 30.928341108151987 -0.0018262913863015125]  CenterOfMassUnits=mm  MomentsOfInertia=[14.640748377051393 9.6696912582654697 14.640902193857929]  MomentsOfInertiaUnits=kg*mm^2  ProductsOfInertia=[0.0065014820412302417 0 0]  ProductsOfInertiaUnits=kg*mm^2  GraphicType=FromGeometry  MarkerShape=Sphere  MarkerSize=10  GraphicVisPropType=SimpleVisualProperties  GraphicDiffuseColor=[0.53725490196078429 0.34901960784313724 0.33725490196078434]  GraphicOpacity=1  GraphicSpecularColor=[0.5 0.5 0.5 1.0]  GraphicAmbientColor=[0.15 0.15 0.15 1.0]  GraphicEmissiveColor=[0.0 0.0 0.0 1.0]  GraphicShininess=75  DoExposeReferenceFrame=on  SerializedFrames=<Frames/>
  F : PMIOPort  Side=Left
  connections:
  Solid/RConn1 -- ReferenceFrame/RConn1 -- F/RConn1

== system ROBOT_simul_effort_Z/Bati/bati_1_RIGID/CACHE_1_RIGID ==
  ReferenceFrame : sm_lib/Frames and Transforms/Reference Frame
  Solid : sm_lib/Body Elements/File Solid  ExtGeomFileName=/MATLAB Drive/Fichiers_Matlab_sujetA/Fichiers Matlab/STL/CACHE_Defaut_sldprt.STL  UnitType=Custom  ExtGeomFileUnits=mm  StepReaderType=HEX  ExportConvexHullGeometry=off  InertiaType=Custom  BasedOnType=Density  Density=1000  DensityUnits=kg/(m^3)  Mass=0.011182198960412355  MassUnits=kg  CenterOfMass=[4.3076392714328797 208.54208665729635 7.8822671814956502]  CenterOfMassUnits=mm  MomentsOfInertia=[9.7659613803690544 11.857978985199471 3.5448360594417863]  MomentsOfInertiaUnits=kg*mm^2  ProductsOfInertia=[-0.087124917777044883 -0.069374532976861802 0.10473407202046144]  ProductsOfInertiaUnits=kg*mm^2  GraphicType=FromGeometry  MarkerShape=Sphere  MarkerSize=10  GraphicVisPropType=SimpleVisualProperties  GraphicDiffuseColor=[0.75294117647058822 0.75294117647058822 0.75294117647058822]  GraphicOpacity=1  GraphicSpecularColor=[0.5 0.5 0.5 1.0]  GraphicAmbientColor=[0.15 0.15 0.15 1.0]  GraphicEmissiveColor=[0.0 0.0 0.0 1.0]  GraphicShininess=75  DoExposeReferenceFrame=on  SerializedFrames=<Frames/>
  F : PMIOPort  Side=Left
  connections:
  Solid/RConn1 -- ReferenceFrame/RConn1 -- F/RConn1

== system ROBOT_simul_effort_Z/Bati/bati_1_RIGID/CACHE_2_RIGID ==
  ReferenceFrame : sm_lib/Frames and Transforms/Reference Frame
  Solid : sm_lib/Body Elements/File Solid  ExtGeomFileName=/MATLAB Drive/Fichiers_Matlab_sujetA/Fichiers Matlab/STL/CACHE_Defaut_sldprt.STL  UnitType=Custom  ExtGeomFileUnits=mm  StepReaderType=HEX  ExportConvexHullGeometry=off  InertiaType=Custom  BasedOnType=Density  Density=1000  DensityUnits=kg/(m^3)  Mass=0.011182198960412355  MassUnits=kg  CenterOfMass=[4.3076392714328797 208.54208665729635 7.8822671814956502]  CenterOfMassUnits=mm  MomentsOfInertia=[9.7659613803690544 11.857978985199471 3.5448360594417863]  MomentsOfInertiaUnits=kg*mm^2  ProductsOfInertia=[-0.087124917777044883 -0.069374532976861802 0.10473407202046144]  ProductsOfInertiaUnits=kg*mm^2  GraphicType=FromGeometry  MarkerShape=Sphere  MarkerSize=10  GraphicVisPropType=SimpleVisualProperties  GraphicDiffuseColor=[0.75294117647058822 0.75294117647058822 0.75294117647058822]  GraphicOpacity=1  GraphicSpecularColor=[0.5 0.5 0.5 1.0]  GraphicAmbientColor=[0.15 0.15 0.15 1.0]  GraphicEmissiveColor=[0.0 0.0 0.0 1.0]  GraphicShininess=75  DoExposeReferenceFrame=on  SerializedFrames=<Frames/>
  F : PMIOPort  Side=Left
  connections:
  Solid/RConn1 -- ReferenceFrame/RConn1 -- F/RConn1

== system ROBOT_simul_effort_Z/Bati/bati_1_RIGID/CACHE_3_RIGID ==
  ReferenceFrame : sm_lib/Frames and Transforms/Reference Frame
  Solid : sm_lib/Body Elements/File Solid  ExtGeomFileName=/MATLAB Drive/Fichiers_Matlab_sujetA/Fichiers Matlab/STL/CACHE_Defaut_sldprt.STL  UnitType=Custom  ExtGeomFileUnits=mm  StepReaderType=HEX  ExportConvexHullGeometry=off  InertiaType=Custom  BasedOnType=Density  Density=1000  DensityUnits=kg/(m^3)  Mass=0.011182198960412355  MassUnits=kg  CenterOfMass=[4.3076392714328797 208.54208665729635 7.8822671814956502]  CenterOfMassUnits=mm  MomentsOfInertia=[9.7659613803690544 11.857978985199471 3.5448360594417863]  MomentsOfInertiaUnits=kg*mm^2  ProductsOfInertia=[-0.087124917777044883 -0.069374532976861802 0.10473407202046144]  ProductsOfInertiaUnits=kg*mm^2  GraphicType=FromGeometry  MarkerShape=Sphere  MarkerSize=10  GraphicVisPropType=SimpleVisualProperties  GraphicDiffuseColor=[0.75294117647058822 0.75294117647058822 0.75294117647058822]  GraphicOpacity=1  GraphicSpecularColor=[0.5 0.5 0.5 1.0]  GraphicAmbientColor=[0.15 0.15 0.15 1.0]  GraphicEmissiveColor=[0.0 0.0 0.0 1.0]  GraphicShininess=75  DoExposeReferenceFrame=on  SerializedFrames=<Frames/>
  F : PMIOPort  Side=Left
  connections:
  Solid/RConn1 -- ReferenceFrame/RConn1 -- F/RConn1

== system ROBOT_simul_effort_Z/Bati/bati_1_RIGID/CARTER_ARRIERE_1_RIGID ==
  ReferenceFrame : sm_lib/Frames and Transforms/Reference Frame
  Solid : sm_lib/Body Elements/File Solid  ExtGeomFileName=/MATLAB Drive/Fichiers_Matlab_sujetA/Fichiers Matlab/STL/CARTER ARRIERE_Defaut_sldprt.STL  UnitType=Custom  ExtGeomFileUnits=mm  StepReaderType=HEX  ExportConvexHullGeometry=off  InertiaType=Custom  BasedOnType=Density  Density=1000  DensityUnits=kg/(m^3)  Mass=0.12081050845213158  MassUnits=kg  CenterOfMass=[0.027688933623677491 107.2258121438302 -1.1182869436416025]  CenterOfMassUnits=mm  MomentsOfInertia=[436.20873458136924 359.38976174708495 770.46596034318191]  MomentsOfInertiaUnits=kg*mm^2  ProductsOfInertia=[18.068269630416292 -0.016904145152124985 0.032703140147255623]  ProductsOfInertiaUnits=kg*mm^2  GraphicType=FromGeometry  MarkerShape=Sphere  MarkerSize=10  GraphicVisPropType=SimpleVisualProperties  GraphicDiffuseColor=[1 1 1]  GraphicOpacity=1  GraphicSpecularColor=[0.5 0.5 0.5 1.0]  GraphicAmbientColor=[0.15 0.15 0.15 1.0]  GraphicEmissiveColor=[0.0 0.0 0.0 1.0]  GraphicShininess=75  DoExposeReferenceFrame=on  SerializedFrames=<Frames/>
  F : PMIOPort  Side=Left
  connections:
  Solid/RConn1 -- ReferenceFrame/RConn1 -- F/RConn1

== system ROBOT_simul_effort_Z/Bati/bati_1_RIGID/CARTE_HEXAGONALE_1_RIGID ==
  ReferenceFrame : sm_lib/Frames and Transforms/Reference Frame
  Solid : sm_lib/Body Elements/File Solid  ExtGeomFileName=/MATLAB Drive/Fichiers_Matlab_sujetA/Fichiers Matlab/STL/CARTE HEXAGONALE_Defaut_sldprt.STL  UnitType=Custom  ExtGeomFileUnits=mm  StepReaderType=HEX  ExportConvexHullGeometry=off  InertiaType=Custom  BasedOnType=Density  Density=1000  DensityUnits=kg/(m^3)  Mass=0.026994433881078982  MassUnits=kg  CenterOfMass=[-1.609455224288012 -0.90517012664311758 2.5720012204185174]  CenterOfMassUnits=mm  MomentsOfInertia=[28.923221067904205 24.898136547803855 53.038824077161053]  MomentsOfInertiaUnits=kg*mm^2  ProductsOfInertia=[0.34251255903735656 0.14956628541838315 1.4697500359655211]  ProductsOfInertiaUnits=kg*mm^2  GraphicType=FromGeometry  MarkerShape=Sphere  MarkerSize=10  GraphicVisPropType=SimpleVisualProperties  GraphicDiffuseColor=[0 0.50196078431372548 0]  GraphicOpacity=1  GraphicSpecularColor=[0.5 0.5 0.5 1.0]  GraphicAmbientColor=[0.15 0.15 0.15 1.0]  GraphicEmissiveColor=[0.0 0.0 0.0 1.0]  GraphicShininess=75  DoExposeReferenceFrame=on  SerializedFrames=<Frames/>
  F : PMIOPort  Side=Left
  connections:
  Solid/RConn1 -- ReferenceFrame/RConn1 -- F/RConn1

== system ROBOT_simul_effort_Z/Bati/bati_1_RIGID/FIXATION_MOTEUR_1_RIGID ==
  ReferenceFrame : sm_lib/Frames and Transforms/Reference Frame
  Solid : sm_lib/Body Elements/File Solid  ExtGeomFileName=/MATLAB Drive/Fichiers_Matlab_sujetA/Fichiers Matlab/STL/FIXATION MOTEUR_Defaut_sldprt.STL  UnitType=Custom  ExtGeomFileUnits=mm  StepReaderType=HEX  ExportConvexHullGeometry=off  InertiaType=Custom  BasedOnType=Density  Density=1000  DensityUnits=kg/(m^3)  Mass=0.00025251914881442344  MassUnits=kg  CenterOfMass=[0 10.662239702438894 0]  CenterOfMassUnits=mm  MomentsOfInertia=[0.012730499644358427 0.059038940284933263 0.070228178640671796]  MomentsOfInertiaUnits=kg*mm^2  ProductsOfInertia=[0 0 0]  ProductsOfInertiaUnits=kg*mm^2  GraphicType=FromGeometry  MarkerShape=Sphere  MarkerSize=10  GraphicVisPropType=SimpleVisualProperties  GraphicDiffuseColor=[0.792156862745098 0.81960784313725488 0.93333333333333335]  GraphicOpacity=1  GraphicSpecularColor=[0.5 0.5 0.5 1.0]  GraphicAmbientColor=[0.15 0.15 0.15 1.0]  GraphicEmissiveColor=[0.0 0.0 0.0 1.0]  GraphicShininess=75  DoExposeReferenceFrame=on  SerializedFrames=<Frames/>
  F : PMIOPort  Side=Left
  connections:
  Solid/RConn1 -- ReferenceFrame/RConn1 -- F/RConn1

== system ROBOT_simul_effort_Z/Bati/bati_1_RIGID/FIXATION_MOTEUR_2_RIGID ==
  ReferenceFrame : sm_lib/Frames and Transforms/Reference Frame
  Solid : sm_lib/Body Elements/File Solid  ExtGeomFileName=/MATLAB Drive/Fichiers_Matlab_sujetA/Fichiers Matlab/STL/FIXATION MOTEUR_Defaut_sldprt.STL  UnitType=Custom  ExtGeomFileUnits=mm  StepReaderType=HEX  ExportConvexHullGeometry=off  InertiaType=Custom  BasedOnType=Density  Density=1000  DensityUnits=kg/(m^3)  Mass=0.00025251914881442344  MassUnits=kg  CenterOfMass=[0 10.662239702438894 0]  CenterOfMassUnits=mm  MomentsOfInertia=[0.012730499644358427 0.059038940284933263 0.070228178640671796]  MomentsOfInertiaUnits=kg*mm^2  ProductsOfInertia=[0 0 0]  ProductsOfInertiaUnits=kg*mm^2  GraphicType=FromGeometry  MarkerShape=Sphere  MarkerSize=10  GraphicVisPropType=SimpleVisualProperties  GraphicDiffuseColor=[0.792156862745098 0.81960784313725488 0.93333333333333335]  GraphicOpacity=1  GraphicSpecularColor=[0.5 0.5 0.5 1.0]  GraphicAmbientColor=[0.15 0.15 0.15 1.0]  GraphicEmissiveColor=[0.0 0.0 0.0 1.0]  GraphicShininess=75  DoExposeReferenceFrame=on  SerializedFrames=<Frames/>
  F : PMIOPort  Side=Left
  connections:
  Solid/RConn1 -- ReferenceFrame/RConn1 -- F/RConn1

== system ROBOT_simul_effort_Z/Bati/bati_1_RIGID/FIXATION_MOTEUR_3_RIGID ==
  ReferenceFrame : sm_lib/Frames and Transforms/Reference Frame
  Solid : sm_lib/Body Elements/File Solid  ExtGeomFileName=/MATLAB Drive/Fichiers_Matlab_sujetA/Fichiers Matlab/STL/FIXATION MOTEUR_Defaut_sldprt.STL  UnitType=Custom  ExtGeomFileUnits=mm  StepReaderType=HEX  ExportConvexHullGeometry=off  InertiaType=Custom  BasedOnType=Density  Density=1000  DensityUnits=kg/(m^3)  Mass=0.00025251914881442344  MassUnits=kg  CenterOfMass=[0 10.662239702438894 0]  CenterOfMassUnits=mm  MomentsOfInertia=[0.012730499644358427 0.059038940284933263 0.070228178640671796]  MomentsOfInertiaUnits=kg*mm^2  ProductsOfInertia=[0 0 0]  ProductsOfInertiaUnits=kg*mm^2  GraphicType=FromGeometry  MarkerShape=Sphere  MarkerSize=10  GraphicVisPropType=SimpleVisualProperties  GraphicDiffuseColor=[0.792156862745098 0.81960784313725488 0.93333333333333335]  GraphicOpacity=1  GraphicSpecularColor=[0.5 0.5 0.5 1.0]  GraphicAmbientColor=[0.15 0.15 0.15 1.0]  GraphicEmissiveColor=[0.0 0.0 0.0 1.0]  GraphicShininess=75  DoExposeReferenceFrame=on  SerializedFrames=<Frames/>
  F : PMIOPort  Side=Left
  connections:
  Solid/RConn1 -- ReferenceFrame/RConn1 -- F/RConn1

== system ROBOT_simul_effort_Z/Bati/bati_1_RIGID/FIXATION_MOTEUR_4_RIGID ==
  ReferenceFrame : sm_lib/Frames and Transforms/Reference Frame
  Solid : sm_lib/Body Elements/File Solid  ExtGeomFileName=/MATLAB Drive/Fichiers_Matlab_sujetA/Fichiers Matlab/STL/FIXATION MOTEUR_Defaut_sldprt.STL  UnitType=Custom  ExtGeomFileUnits=mm  StepReaderType=HEX  ExportConvexHullGeometry=off  InertiaType=Custom  BasedOnType=Density  Density=1000  DensityUnits=kg/(m^3)  Mass=0.00025251914881442344  MassUnits=kg  CenterOfMass=[0 10.662239702438894 0]  CenterOfMassUnits=mm  MomentsOfInertia=[0.012730499644358427 0.059038940284933263 0.070228178640671796]  MomentsOfInertiaUnits=kg*mm^2  ProductsOfInertia=[0 0 0]  ProductsOfInertiaUnits=kg*mm^2  GraphicType=FromGeometry  MarkerShape=Sphere  MarkerSize=10  GraphicVisPropType=SimpleVisualProperties  GraphicDiffuseColor=[0.792156862745098 0.81960784313725488 0.93333333333333335]  GraphicOpacity=1  GraphicSpecularColor=[0.5 0.5 0.5 1.0]  GraphicAmbientColor=[0.15 0.15 0.15 1.0]  GraphicEmissiveColor=[0.0 0.0 0.0 1.0]  GraphicShininess=75  DoExposeReferenceFrame=on  SerializedFrames=<Frames/>
  F : PMIOPort  Side=Left
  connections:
  Solid/RConn1 -- ReferenceFrame/RConn1 -- F/RConn1

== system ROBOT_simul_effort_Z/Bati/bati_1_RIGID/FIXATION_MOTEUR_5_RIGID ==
  ReferenceFrame : sm_lib/Frames and Transforms/Reference Frame
  Solid : sm_lib/Body Elements/File Solid  ExtGeomFileName=/MATLAB Drive/Fichiers_Matlab_sujetA/Fichiers Matlab/STL/FIXATION MOTEUR_Defaut_sldprt.STL  UnitType=Custom  ExtGeomFileUnits=mm  StepReaderType=HEX  ExportConvexHullGeometry=off  InertiaType=Custom  BasedOnType=Density  Density=1000  DensityUnits=kg/(m^3)  Mass=0.00025251914881442344  MassUnits=kg  CenterOfMass=[0 10.662239702438894 0]  CenterOfMassUnits=mm  MomentsOfInertia=[0.012730499644358427 0.059038940284933263 0.070228178640671796]  MomentsOfInertiaUnits=kg*mm^2  ProductsOfInertia=[0 0 0]  ProductsOfInertiaUnits=kg*mm^2  GraphicType=FromGeometry  MarkerShape=Sphere  MarkerSize=10  GraphicVisPropType=SimpleVisualProperties  GraphicDiffuseColor=[0.792156862745098 0.81960784313725488 0.93333333333333335]  GraphicOpacity=1  GraphicSpecularColor=[0.5 0.5 0.5 1.0]  GraphicAmbientColor=[0.15 0.15 0.15 1.0]  GraphicEmissiveColor=[0.0 0.0 0.0 1.0]  GraphicShininess=75  DoExposeReferenceFrame=on  SerializedFrames=<Frames/>
  F : PMIOPort  Side=Left
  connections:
  Solid/RConn1 -- ReferenceFrame/RConn1 -- F/RConn1

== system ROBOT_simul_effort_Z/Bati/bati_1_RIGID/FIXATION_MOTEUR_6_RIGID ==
  ReferenceFrame : sm_lib/Frames and Transforms/Reference Frame
  Solid : sm_lib/Body Elements/File Solid  ExtGeomFileName=/MATLAB Drive/Fichiers_Matlab_sujetA/Fichiers Matlab/STL/FIXATION MOTEUR_Defaut_sldprt.STL  UnitType=Custom  ExtGeomFileUnits=mm  StepReaderType=HEX  ExportConvexHullGeometry=off  InertiaType=Custom  BasedOnType=Density  Density=1000  DensityUnits=kg/(m^3)  Mass=0.00025251914881442344  MassUnits=kg  CenterOfMass=[0 10.662239702438894 0]  CenterOfMassUnits=mm  MomentsOfInertia=[0.012730499644358427 0.059038940284933263 0.070228178640671796]  MomentsOfInertiaUnits=kg*mm^2  ProductsOfInertia=[0 0 0]  ProductsOfInertiaUnits=kg*mm^2  GraphicType=FromGeometry  MarkerShape=Sphere  MarkerSize=10  GraphicVisPropType=SimpleVisualProperties  GraphicDiffuseColor=[0.792156862745098 0.81960784313725488 0.93333333333333335]  GraphicOpacity=1  GraphicSpecularColor=[0.5 0.5 0.5 1.0]  GraphicAmbientColor=[0.15 0.15 0.15 1.0]  GraphicEmissiveColor=[0.0 0.0 0.0 1.0]  GraphicShininess=75  DoExposeReferenceFrame=on  SerializedFrames=<Frames/>
  F : PMIOPort  Side=Left
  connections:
  Solid/RConn1 -- ReferenceFrame/RConn1 -- F/RConn1
